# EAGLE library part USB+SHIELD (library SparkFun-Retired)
USB+Shield USB connector with shield pins connectable
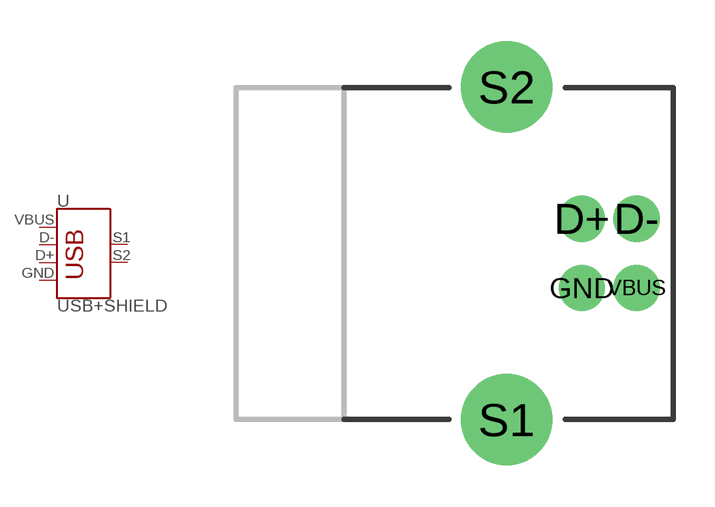
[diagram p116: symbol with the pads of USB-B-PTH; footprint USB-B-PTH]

Designator prefix -

## USB+SHIELD  [USB-B-PTH]
D+  D+
D-  D-
GND  GND  pwr
S1  S1
S2  S2
VBUS  VBUS  pwr

## Footprint USB-B-PTH (pad centres in mm)
USB Type B PTH Mounted Specifications: Pin count:4 main, 2 shield Datasheet referenced for footprint: Example device(s): USB_B
drill 0.914 pad 1.676: D+ 0,1.25; D- 1.981,1.25; GND 0,-1.25; VBUS 1.981,-1.25
drill 2.286: S1 -2.718,-6.02; S2 -2.718,6.02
